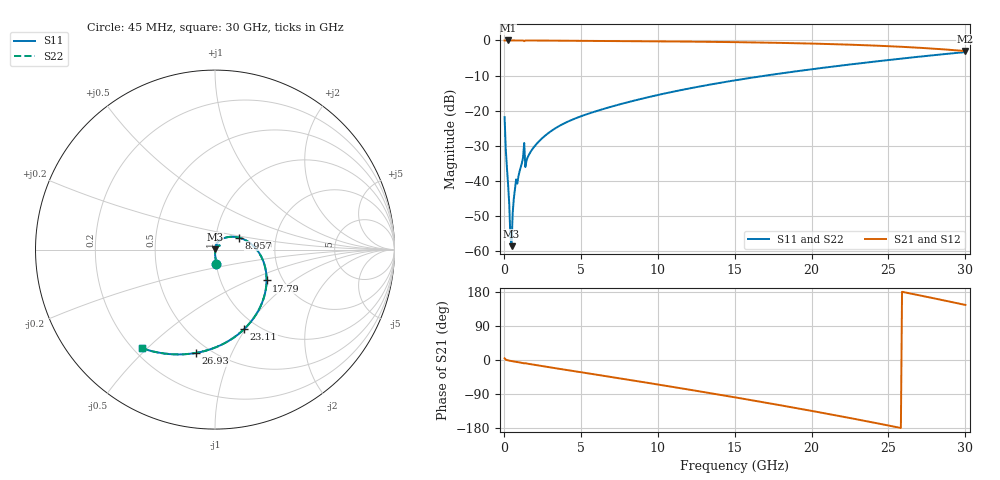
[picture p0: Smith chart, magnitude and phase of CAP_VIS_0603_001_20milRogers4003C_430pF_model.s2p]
! S-parameter model data by Modelithics Inc.  support@modelithics.com  813-866-6335  Tampa FL USA
! S-Parameter data specifications:
! Substrate: 20-mil Rogers 4003C, substrate thickness, H=0.508mm, Dielectric constant, Er=3.75
! PCB Mounting Pad Footprint: Pad width, PadW=0.90mm , Pad length, PadL=1.00mm , Pad gap, PadG (edge-to-edge)=1.00mm , Reference planes=3.0mm apart
! Created Wed Nov 18 13:34:56 2015
# hz S ma R 50
! 2 Port Network Data from SP1.SP block
! freq  magS11  angS11  magS21  angS21  magS12  angS12  magS22  angS22
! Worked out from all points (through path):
!   401 points, 45 MHz to 30 GHz, reference 50 ohm
!   highest |S21| = 0.00 dB at 269.7 MHz (marker M1); lowest = -3.0 dB at 30 GHz (marker M2)
!   group delay of S21, straight-line fit = 19.7 ps
!   lowest |S11| = -58.5 dB at 494.3 MHz (marker M3), VSWR 1.00, Z = 50.1 + j0.107 ohm
!   |S11| at or under -10 dB: start of sweep to 17.01 GHz
!   |S22| runs from -58.5 to -3.3 dB; largest |S21 - S12| = 0
!   S11 on the Smith chart (normalised r, x): 45 MHz: 1.00, -0.16; 8.957 GHz: 1.29, +0.18; 17.79 GHz: 1.65, -0.64; 23.11 GHz: 0.86, -0.99; 26.93 GHz: 0.42, -0.74; 30 GHz: 0.23, -0.48
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4.5e7  0.08103 -85.5  0.9965 4.4  0.9965 4.4  0.08103 -85.5
1.94775e8  0.01562 -89.0  0.9996 -0.2  0.9996 -0.2  0.01562 -89.0
2.696625e8  0.009074 -88.7  0.9996 -1.0  0.9996 -1.0  0.009074 -88.7
3.4455e8  0.004809 -86.9  0.9996 -1.6  0.9996 -1.6  0.004809 -86.9
4.194375e8  0.001627 -77.0  0.9995 -2.2  0.9995 -2.2  0.001627 -77.0
4.94325e8  0.001189 64.3  0.9995 -2.8  0.9995 -2.8  0.001189 64.3
5.692125e8  0.003476 78.4  0.9994 -3.3  0.9994 -3.3  0.003476 78.4
7.93875e8  0.0106 77.9  0.9986 -5.0  0.9986 -5.0  0.0106 77.9
1.168312e9  0.01806 79.6  0.9988 -7.5  0.9988 -7.5  0.01806 79.6
1.54275e9  0.02176 77.6  0.9986 -9.7  0.9986 -9.7  0.02176 77.6
2.066962e9  0.03272 74.2  0.9979 -13.3  0.9979 -13.3  0.03272 74.2
2.965612e9  0.04959 67.1  0.9953 -19.2  0.9953 -19.2  0.04959 67.1
5.062462e9  0.08433 50.6  0.9861 -32.7  0.9861 -32.7  0.08433 50.6
8.956612e9  0.1483 27.0  0.9745 -57.7  0.9745 -57.7  0.1483 27.0
1.007992e10  0.169 20.1  0.9707 -65.1  0.9707 -65.1  0.169 20.1
1.50225e10  0.2709 -11.8  0.9461 -98.6  0.9461 -98.6  0.2709 -11.8
1.779334e10  0.3348 -30.9  0.9248 -118.1  0.9248 -118.1  0.3348 -30.9
2.003996e10  0.3902 -47.0  0.9023 -134.5  0.9023 -134.5  0.3902 -47.0
2.311035e10  0.4722 -70.0  0.8616 -157.9  0.8616 -157.9  0.4722 -70.0
2.505742e10  0.5284 -85.3  0.828 -173.3  0.828 -173.3  0.5284 -85.3
2.692961e10  0.5855 -100.5  0.7885 171.4  0.7885 171.4  0.5855 -100.5
3e10  0.683 -126.4  0.7061 145.3  0.7061 145.3  0.683 -126.4
